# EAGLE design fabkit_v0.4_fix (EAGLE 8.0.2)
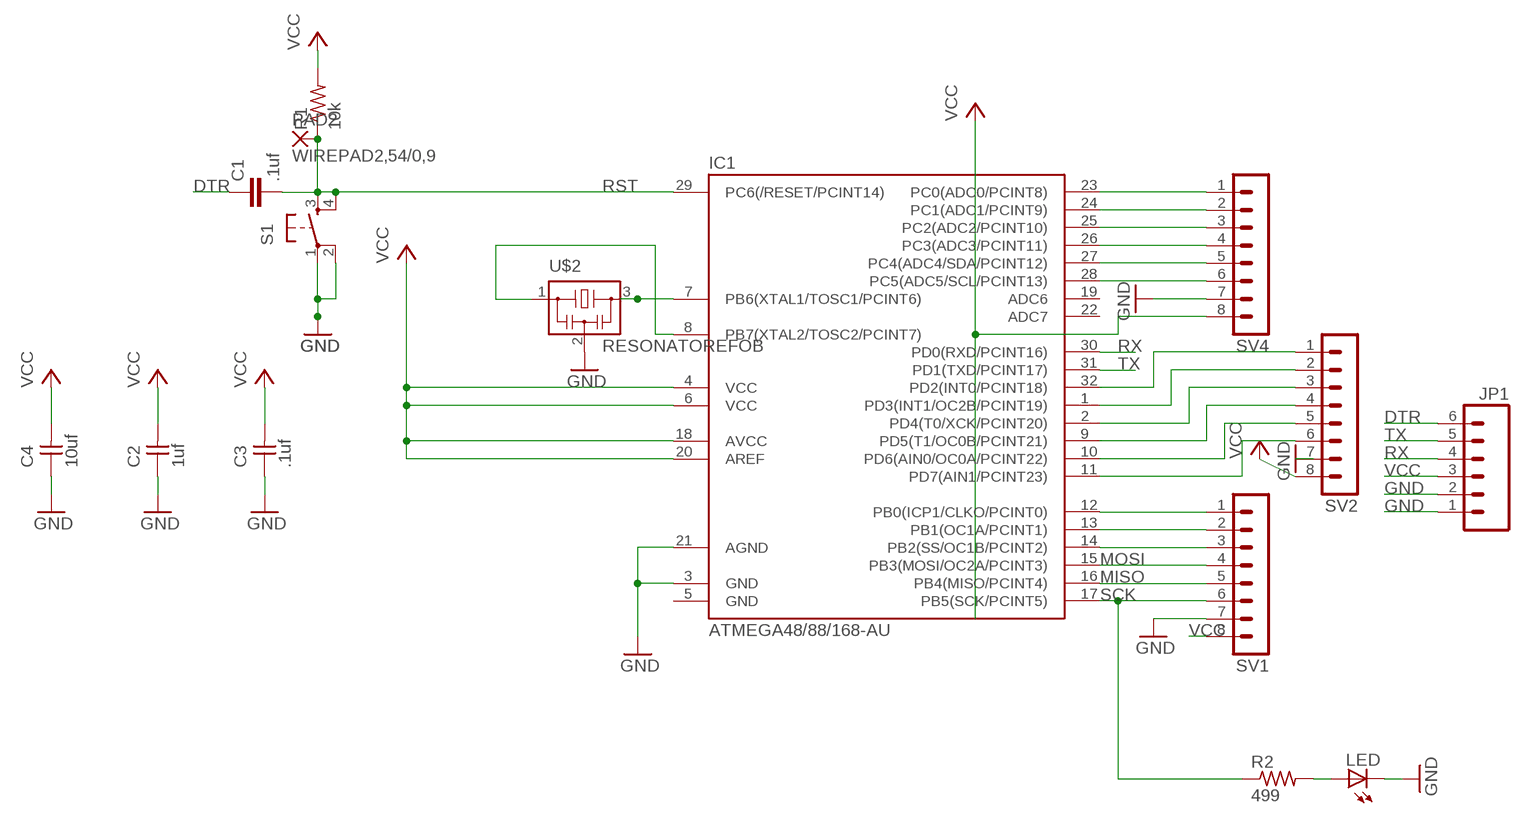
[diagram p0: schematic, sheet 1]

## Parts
C1  .1uf  C-EUC1206  [C1206]
C2  1uf  UNPOLARIZED_CAPACITOR1206  [1206]
C3  .1uf  UNPOLARIZED_CAPACITOR1206  [1206]
C4  10uf  UNPOLARIZED_CAPACITOR1206  [1206]
IC1  ATMEGA48/88/168-AU  [TQFP32-08]
JP1  M06SMD  [1X06-SMD]
LED  LED1206  [1206]
PAD2  WIREPAD2,54/0,9  [2,54/0,9]
R1  10k  RESISTOR1206  [1206]
R2  499  RESISTOR1206  [1206]
S1  6MM_SWITCH6MM_SWITCH  [6MM_SWITCH]
SV1  MA08-1  [MA08-1]
SV2  MA08-1  [MA08-1]
SV4  MA08-1  [MA08-1]
U$2  RESONATOREFOB  [EFOBM]

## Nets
DTR: C1.1 JP1.6
GND: C2.1 C3.1 C4.1 IC1.3(GND) IC1.21(AGND) JP1.1 JP1.2 LED.2(C) S1.1(P) S1.2(P1) SV1.7 SV2.7 SV4.7 U$2.2
MISO: IC1.16(PB4(MISO/PCINT4)) SV1.5
MOSI: IC1.15(PB3(MOSI/OC2A/PCINT3)) SV1.4
N$1: IC1.8(PB7(XTAL2/TOSC2/PCINT7)) U$2.1
N$9: IC1.7(PB6(XTAL1/TOSC1/PCINT6)) U$2.3
N$23: LED.1(A) R2.2
PB0: IC1.12(PB0(ICP1/CLKO/PCINT0)) SV1.1
PB1: IC1.13(PB1(OC1A/PCINT1)) SV1.2
PB2: IC1.14(PB2(SS/OC1B/PCINT2)) SV1.3
PC0: IC1.23(PC0(ADC0/PCINT8)) SV4.1
PC1: IC1.24(PC1(ADC1/PCINT9)) SV4.2
PC2: IC1.25(PC2(ADC2/PCINT10)) SV4.3
PC3: IC1.26(PC3(ADC3/PCINT11)) SV4.4
PC4: IC1.27(PC4(ADC4/SDA/PCINT12)) SV4.5
PC5: IC1.28(PC5(ADC5/SCL/PCINT13)) SV4.6
PD2: IC1.32(PD2(INT0/PCINT18)) SV2.1
PD3: IC1.1(PD3(INT1/OC2B/PCINT19)) SV2.2
PD4: IC1.2(PD4(T0/XCK/PCINT20)) SV2.3
PD5: IC1.9(PD5(T1/OC0B/PCINT21)) SV2.4
PD6: IC1.10(PD6(AIN0/OC0A/PCINT22)) SV2.5
PD7: IC1.11(PD7(AIN1/PCINT23)) SV2.6
RST: C1.2 IC1.29(PC6(/RESET/PCINT14)) PAD2.1(P) R1.1 S1.3(S) S1.4(S1)
RX: IC1.30(PD0(RXD/PCINT16)) JP1.4
SCK: IC1.17(PB5(SCK/PCINT5)) R2.1 SV1.6
TX: IC1.31(PD1(TXD/PCINT17)) JP1.5
VCC: C2.2 C3.2 C4.2 IC1.4(VCC) IC1.6(VCC) IC1.18(AVCC) IC1.20(AREF) JP1.3 R1.2 SV1.8 SV2.8 SV4.8
Unconnected: IC1.19(ADC6) IC1.22(ADC7)

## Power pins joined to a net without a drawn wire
GND: IC1.5(GND)

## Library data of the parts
C1 = rcl:C-EU: CAPACITOR, European symbol
C2-C4 = ng:UNPOLARIZED_CAPACITOR: unpolarized_capacitor
IC1 = atmega8:ATMEGA48/88/168
JP1 = SparkFun:M06: Header 6 Standard 6-pin 0.1" header. Use with straight break away headers (SKU : PRT-00116), right angle break away headers (PRT-00553), swiss pins (PRT-00743), machine pins (PRT-00117), and female headers (PRT-00115). Molex polarized connector foot print use with SKU : PRT-08094 with associated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
LED = ng:LED
PAD2 = wirepad:WIREPAD: Wire PAD connect wire on PCB
R1 R2 = ng:RESISTOR
S1 = ng:6MM_SWITCH: OMRON SWITCH
SV1 SV2 SV4 = con-lstb:MA08-1: PIN HEADER
U$2 = fab:RESONATOR

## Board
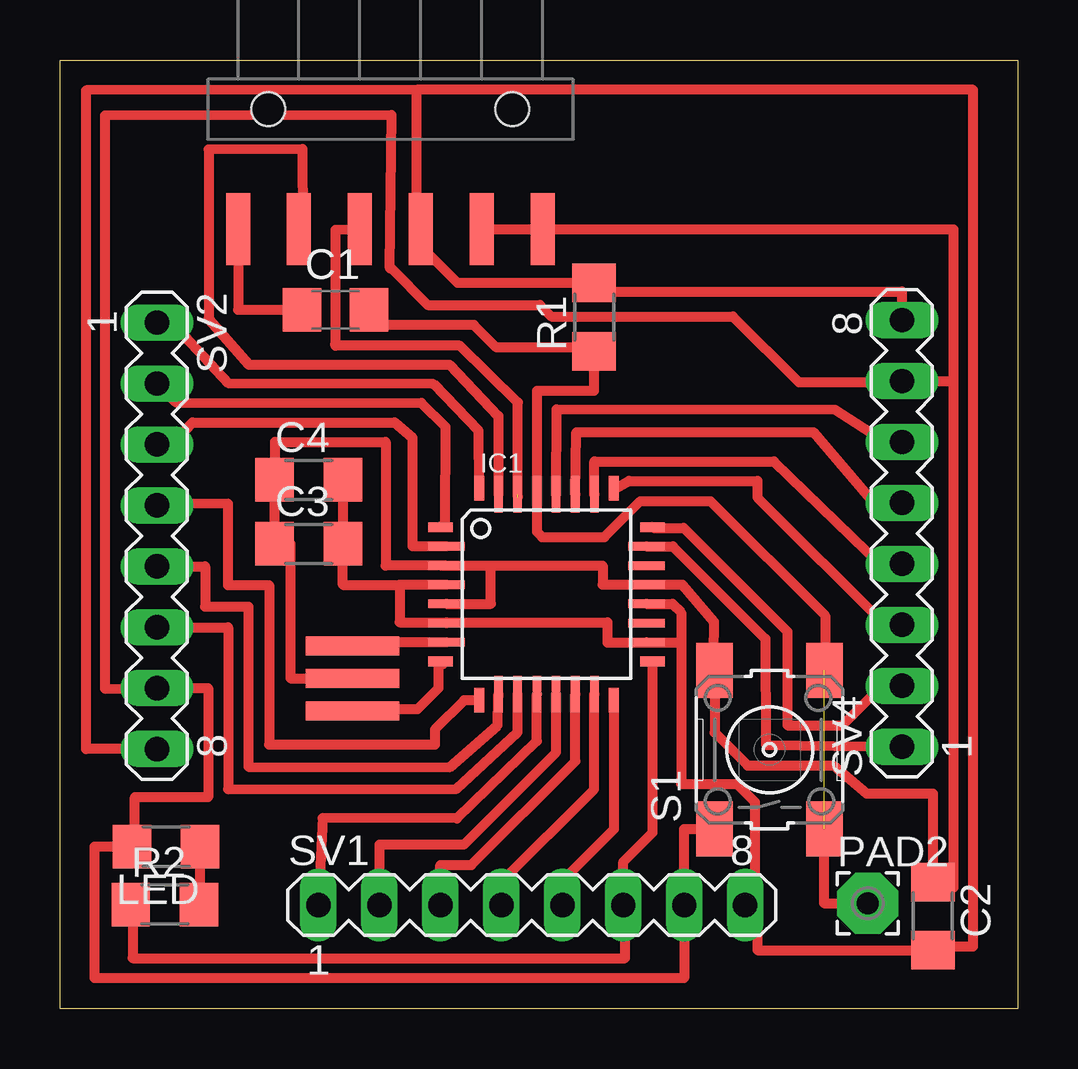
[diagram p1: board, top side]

Size 39.9 x 39.55 mm. Coordinates in mm from the lower left corner, seen from the top.
Outline: 0,39.55 39.9,39.55 39.9,0 0,0 0,39.55
Copper layers (1*16): Top 0.035mm / dielectric 1.5mm / Bottom 0.035mm
Design rules "default *": minimum track width 10mil, minimum drill 24mil, track to track 16mil, track to pad 16mil, pad to pad 16mil, via to via 16mil, smd to smd 16mil, copper to edge 16mil, drill to drill 8mil, minimum pad ring 10mil, minimum via ring 8mil, stop-mask expansion 4mil, vias tented up to drill 0mil, thermal gap 10mil

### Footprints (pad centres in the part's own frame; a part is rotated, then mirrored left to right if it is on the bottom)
C1206 = smd 1.6 x 1.8: 1 -1.4,0; 2 1.4,0
1206 = smd 1.6 x 1.803: 1 -1.422,0; 2 1.422,0
TQFP32-08 = smd 1.016 x 0.406: 1 -4.42,2.8; 8 -4.42,-2.8; 17 4.42,-2.8; 24 4.42,2.8 | smd 1.524 x 0.356: 2 -4.166,2; 3 -4.166,1.2; 4 -4.166,0.4; 5 -4.166,-0.4; 6 -4.166,-1.2; 7 -4.166,-2; 18 4.166,-2; 19 4.166,-1.2; 20 4.166,-0.4; 21 4.166,0.4; 22 4.166,1.2; 23 4.166,2 | smd 0.406 x 1.016: 9 -2.8,-4.42; 16 2.8,-4.42; 25 2.8,4.42; 32 -2.8,4.42 | smd 0.356 x 1.524: 10 -2,-4.166; 11 -1.2,-4.166; 12 -0.4,-4.166; 13 0.4,-4.166; 14 1.2,-4.166; 15 2,-4.166; 26 2,4.166; 27 1.2,4.166; 28 0.4,4.166; 29 -0.4,4.166; 30 -1.2,4.166; 31 -2,4.166
1X06-SMD = smd 1 x 3: 1 -6.35,5; 2 -3.81,5; 3 -1.27,5; 4 1.27,5; 5 3.81,5; 6 6.35,5 | hole 1.4: -5.08,0; 5.08,0
2,54/0,9 = drill 0.914 pad 2.54 octagon: 1 0,0
6MM_SWITCH = smd 2.286 x 1.524: 1 -3.302,2.286; 2 3.302,2.286; 3 -3.302,-2.286; 4 3.302,-2.286
MA08-1 = drill 1.016 long: 1 -8.89,0; 2 -6.35,0; 3 -3.81,0; 4 -1.27,0; 5 1.27,0; 6 3.81,0; 7 6.35,0; 8 8.89,0
EFOBM = smd 0.8 x 3.9: 1 -1.35,0; 2 0,0; 3 1.35,0

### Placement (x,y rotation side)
C1  11.48,29.13 0 top
C2  36.37,3.86 270 top
C3  10.36,19.38 0 top
C4  10.36,22.05 0 top
IC1  20.27,17.27 0 top
JP1  13.77,37.49 180 top
LED  4.42,6.76 180 top
PAD2  33.66,4.39 0 top
R1  22.25,28.83 90 top
R2  4.37,4.34 0 top
S1  29.57,10.79 90 top
SV1  19.66,4.32 0 top
SV2  4.04,19.71 270 top
SV4  35.08,19.81 90 top
U$2  12.19,13.77 90 top

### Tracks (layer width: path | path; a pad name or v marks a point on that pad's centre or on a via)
DTR
  Top 0.406: JP1.6 7.42,29.13 C1.1
GND
  Top 0.356: 24.33,17.68 24.33,17.67 IC1.21
  Top 0.406: 15.9,18.47 15.88,18.47 | 15.9,18.47 17.96,18.47 | 15.9,18.47 15.93,18.47 | 15.93,18.47 IC1.3 13.56,18.47 13.56,23.62 8.97,23.62 8.97,22.07 C4.1 C3.1 9.6,19.38 9.6,13.77 U$2.2 | 15.93,18.47 | JP1.2 JP1.1 37.24,32.49 37.24,26.16 | 17.96,18.47 22.61,18.47 22.61,17.68 IC1.21 25.94,17.67 27.25,16.13 27.23,13.51 S1.2 27.28,11.51 28.65,10.13 32.23,10.13 33.6,8.97 36.37,8.97 C2.1 36.27,5.05 37.24,5.05 37.24,26.16 | IC1.5 17.96,16.87 17.96,18.47 | 37.24,26.16 SV4.7 35.03,26.11 30.79,26.11 28.04,28.85 20.47,28.85 19.99,29.34 15.32,29.34 13.79,30.86 13.74,30.86 13.82,37.26 1.88,37.24 1.88,13.34 SV2.7 6.17,13.36 6.17,8.81 3.12,8.81 3.12,6.88 LED.2 1.45,6.76 1.45,1.27 26.01,1.27 SV1.7 26.01,7.49 S1.1
MISO
  Top 0.406: SV1.5 20.93,5.33 23.09,7.49 23.09,12.83 IC1.16
MOSI
  Top 0.406: SV1.4 18.39,5.28 22.25,9.14 22.25,13.09 IC1.15
N$1
  Top 0.406: 15.95,14.37 IC1.8 15.77,14.4 15.77,13.36 14.91,12.49 12.19,12.49 U$2.1
N$9
  Top 0.406: IC1.7 12.35,15.27 arc90 U$2.3
N$23
  Top 0.406: R2.2 5.97,4.34 5.84,4.47 LED.1
PB0
  Top 0.406: SV1.1 10.95,7.95 16.54,7.92 19.87,11.16 IC1.12
PB1
  Top 0.406: SV1.2 13.31,6.83 16.82,6.83 20.67,10.69 IC1.13
PB2
  Top 0.406: SV1.3 15.85,5.99 17.14,5.99 21.47,10.32 IC1.14
PC0
  Top 0.406: IC1.23 25.53,19.27 29.39,15.42 29.41,11 SV4.1
PC1
  Top 0.406: 24.64,20.07 IC1.24 24.72,20.04 25.98,20.04 30.3,15.72 30.3,11.81 32.59,11.81 34.19,13.41 35.03,13.41 SV4.2
PC2
  Top 0.406: IC1.25 23.16,21.69 23.7,22 29.06,22 29.06,21.31 34.42,15.95 35.03,15.95 SV4.3
PC3
  Top 0.406: 22.25,21.44 IC1.26 22.27,22.81 29.74,22.81 34.27,18.44 34.98,18.44 SV4.4
PC4
  Top 0.406: IC1.27 21.52,24.03 31.39,24.03 34.01,20.95 34.95,20.95 SV4.5
PC5
  Top 0.406: IC1.28 20.7,24.99 32.28,24.97 34.39,23.62 SV4.6
PD2
  Top 0.406: IC1.32 17.44,24.09 15.57,26.04 7.04,26.06 4.67,28.6 SV2.1
PD3
  Top 0.406: SV2.2 4.83,25.27 15.06,25.25 16.05,24.26 16.03,20.25 IC1.1
PD4
  Top 0.406: SV2.3 4.65,23.52 5.51,24.43 13.95,24.43 14.68,23.8 14.68,19.28 IC1.2
PD5
  Top 0.406: 17.47,12.64 IC1.9 16.84,12.85 15.62,11.63 15.62,11 8.71,11 8.71,17.65 7.01,17.65 7.01,21.06 4.04,21.03 SV2.4
PD6
  Top 0.406: SV2.5 6.04,18.44 6.04,16.76 7.85,16.76 7.85,10.08 16.23,10.06 18.24,11.81 18.26,13.02 IC1.10
PD7
  Top 0.406: IC1.11 19.07,11.53 16.54,9.17 7.01,9.14 7.01,15.9 SV2.6
RST  (1 unrouted)
  Top 0.406: S1.3 31.83,7.49 31.83,4.39 PAD2.1 | C1.2 13.52,28.5 17.25,28.5 18.19,27.56 22.1,27.56 R1.1 22.25,25.76 19.87,25.76 IC1.29 19.87,19.88 20.09,19.66 22.68,19.66 24.18,21.16 27.1,21.16 31.88,16.38 31.88,14.12 S1.4
RX  (1 unrouted)
  Top 0.406: 12.52,32.29 12.52,32.61 12.62,32.77 12.5,32.28 12.65,32.9 JP1.4 11.48,32.47 11.48,27.64 | 19.07,21.34 19.07,25.27 16.66,27.64 11.48,27.64 | 11.46,27.69 11.48,27.64
SCK
  Top 0.305: 23.55,4.32 SV1.6
  Top 0.406: R2.1 3.02,3.63 3.02,2.11 23.55,2.11 23.55,4.32 | SV1.6 23.47,6.12 24.69,7.34 IC1.17
TX
  Top 0.406: JP1.5 10.13,32.59 10.11,35.84 6.2,35.81 6.2,28.75 7.87,26.85 16.23,26.85 18.26,24.71 18.26,21.48 IC1.31
VCC
  Top 0.254: 21.64,30.18 21.79,30.05 R1.2 | 14.86,32.69 JP1.3 15.19,32.69 | 1.32,38.3 1.09,38.28
  Top 0.305: IC1.20
  Top 0.406: 15.14,32.52 JP1.3 15.02,31.98 15.01,31.8 16.57,30.25 R1.2 22.61,29.9 35.08,29.9 SV4.8 | 21.77,30.2 21.64,30.18 21.61,30.2 | IC1.4 14.15,17.67 | 14.15,17.67 14.15,16.1 16.1,16.1 | 16.1,16.1 IC1.6 | 16.1,16.1 22.81,16.1 22.81,15.27 IC1.18 25.88,15.27 | 25.88,15.27 25.88,9.37 28.19,9.37 28.96,8.61 28.96,4.72 SV1.8 28.55,4.27 29.06,4.27 29.06,2.44 C2.2 36.45,2.59 38.05,2.59 38.05,38.3 14.86,38.3 | SV2.8 1.09,10.82 1.09,38.28 14.86,38.3 | 14.86,32.69 14.86,38.3 | 14.15,17.67 11.79,17.67 C3.2 C4.2 | IC1.20 25.52,16.87 25.88,16.51 25.88,15.27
